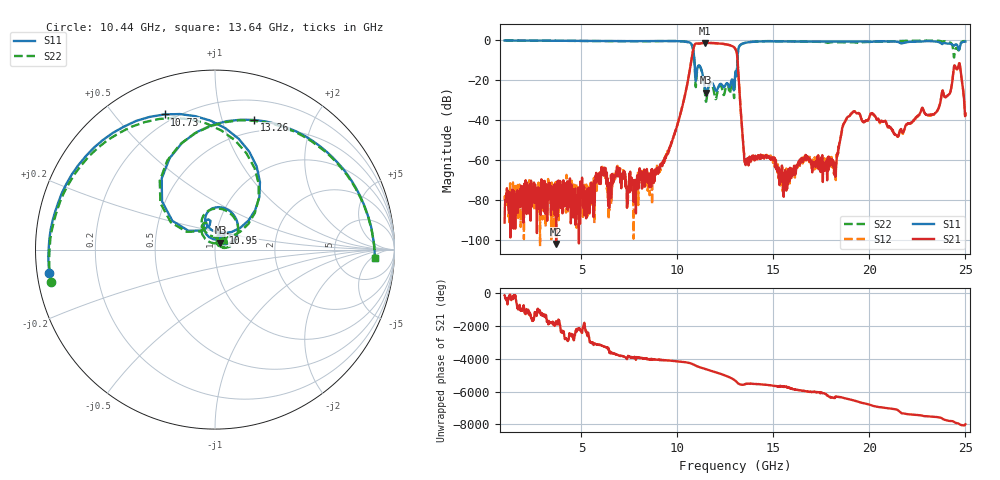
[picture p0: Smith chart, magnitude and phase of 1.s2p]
!The following data was pulled from an Agilent PNA
!This sNp file was generated from the data in the RF Test software
!NOTE:  Smoothing/Math/Corrections applied on any given trace ARE included in the data saved here
# MHz S dB R 50
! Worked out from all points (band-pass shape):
!   1601 points, 1 GHz to 25 GHz, reference 50 ohm
!   highest |S21| = -1.21 dB at 11.46 GHz (marker M1); lowest = -102.1 dB at 3.685 GHz (marker M2)
!   |S21| within 3 dB of the highest: 10.83 GHz to 13.02 GHz (2.184 GHz wide, 18.3 % of centre)
!   lowest |S11| = -26.2 dB at 11.5 GHz (marker M3), VSWR 1.10, Z = 53 + j4.06 ohm
!   |S11| at or under -10 dB: 10.88 GHz to 13.12 GHz (2.24 GHz wide, 18.7 % of centre)
!   |S22| runs from -30.7 to 0.0 dB; largest |S21 - S12| = 0.012
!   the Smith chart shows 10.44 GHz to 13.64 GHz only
!   S11 on the Smith chart (normalised r, x): 10.44 GHz: 0.03, -0.07; 10.73 GHz: 0.16, +0.68; 10.95 GHz: 1.08, +0.20; 13.26 GHz: 0.38, +1.28; 13.64 GHz: 14, -7
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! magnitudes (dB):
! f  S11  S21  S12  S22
! 1 GHz  0.0  -91.4  -80.0  0.0
! 3.685 GHz  -0.1  -102.1  -71.6  -0.2
! 5.005 GHz  -0.2  -76.0  -77.5  -0.2
! 6.085 GHz  -0.3  -66.3  -63.3  -0.4
! 9.01 GHz  -0.3  -64.9  -65.2  -0.3
! 10.44 GHz  -0.6  -25.5  -25.6  -0.6
! 10.73 GHz  -1.9  -9.5  -9.5  -2.0
! 10.95 GHz  -19.7  -1.6  -1.6  -22.5
! 11.46 GHz  -25.1  -1.2  -1.2  -28.7
! 11.5 GHz  -26.2  -1.2  -1.2  -30.7
! 13 GHz  -17.8  -4.0  -4.0  -19.2
! 13.26 GHz  -2.4  -28.9  -29.0  -2.5
! 13.46 GHz  -1.3  -56.0  -56.4  -1.4
! 13.64 GHz  -1.0  -60.4  -59.6  -1.0
! 15.62 GHz  -0.5  -66.2  -67.2  -0.4
! 17 GHz  -0.6  -61.9  -62.3  -0.7
! 18.19 GHz  -0.5  -63.0  -66.9  -0.8
! 19.15 GHz  -0.5  -35.8  -35.9  -0.9
! 21.01 GHz  -0.5  -43.6  -43.5  -0.5
! 23.43 GHz  -0.5  -36.4  -36.7  -0.1
! 24.58 GHz  -2.5  -14.2  -14.4  -4.2
! 25 GHz  -0.6  -36.6  -36.4  -0.5
